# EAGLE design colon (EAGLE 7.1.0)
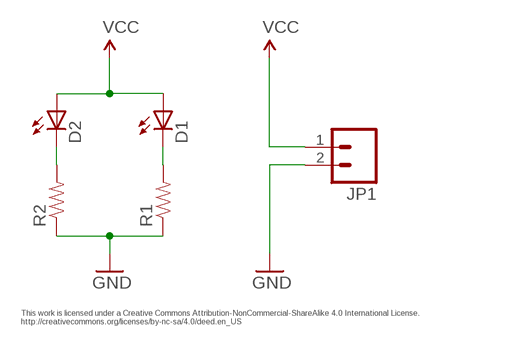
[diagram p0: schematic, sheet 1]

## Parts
D1  LED-RED1206  [LED-1206]
D2  LED-RED1206  [LED-1206]
JP1  M021X02_NO_SILK  [1X02_NO_SILK]
R1  RESISTOR0805-RES  [0805]
R2  RESISTOR0805-RES  [0805]

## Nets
GND: JP1.2 R1.1 R2.1
N$1: D2.C R2.2
N$2: D1.C R1.2
VCC: D1.A D2.A JP1.1

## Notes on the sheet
- This work is licensed under a Creative Commons Attribution-NonCommercial-ShareAlike 4.0 International License.
  http://creativecommons.org/licenses/by-nc-sa/4.0/deed.en_US

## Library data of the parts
D1 D2 = SparkFun-LED:LED-RED: Assorted Red LEDs; PROD_ID: DIO-00809; VALUE: RED
JP1 = SparkFun-Connectors:M02: Standard 2-pin 0.1" header. Use with
R1 R2 = SparkFun-Resistors:RESISTOR: Resistor

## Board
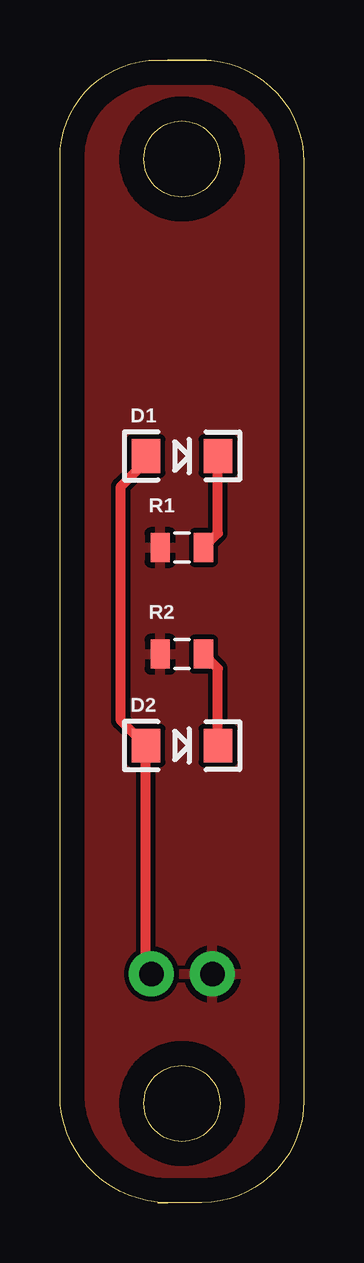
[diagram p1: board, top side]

Size 10.16 x 47.62 mm. Coordinates in mm from the lower left corner, seen from the top.
Outline: 4.49,0 5.9,0 arc90 10.16,4.26 10.16,43.37 arc90 5.9,47.62 4.07,47.62 arc90 0,43.56 0,43.18 0,42.55 0,4.49 arc90 4.49,0
Outline: 4.07,0 4.49,0
Outline: 6.09,47.62 4.49,47.62
Outline: 5.08,45.09 arc-180 5.08,41.91 arc-180 5.08,45.09
Outline: 5.08,2.54 arc-180 5.08,5.71 arc-180 5.08,2.54
Copper layers (1*16): Top 0.035mm / dielectric 1.5mm / Bottom 0.035mm
Design rules "default": minimum track width 10mil, minimum drill 24mil, track to track 8mil, track to pad 8mil, pad to pad 8mil, via to via 8mil, smd to smd 8mil, copper to edge 40mil, drill to drill 8mil, minimum pad ring 10mil, minimum via ring 8mil, stop-mask expansion 4mil, vias tented up to drill 0mil, thermal gap 10mil

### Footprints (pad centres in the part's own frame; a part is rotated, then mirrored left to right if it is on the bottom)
LED-1206 = smd 1.2 x 1.4: A -1.5,0; C 1.5,0
1X02_NO_SILK = drill 1.016 pad 1.88: 1 0,0; 2 2.54,0
0805 = smd 0.8 x 1.2: 1 -0.9,0; 2 0.9,0

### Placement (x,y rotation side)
D1  5.08,31.12 0 top
D2  5.08,19.05 0 top
JP1  3.81,9.53 0 top
R1  5.08,27.3 0 top
R2  5.08,22.86 0 top

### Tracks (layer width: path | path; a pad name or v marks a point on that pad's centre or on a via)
GND
  pour Top: -5.08,50.8 13.97,50.8 13.97,-3.17 -5.08,-3.17
N$1
  Top 0.406: D2.C 6.58,22.26 R2.2
N$2
  Top 0.406: R1.2 6.58,27.91 D1.C
VCC
  Top 0.406: JP1.1 3.58,9.75 D2.A 2.54,20.09 2.54,29.85 3.58,30.89 D1.A

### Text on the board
Unrouted: This work is licensed under a Creative Commons Attribution-NonCommercial-ShareAlike 4.0 International License. / http://creativecommons.org/licenses/by-nc-sa/4.0/deed.en_US
bNames: Kevin Rye, 2015 - V1.0 | Vcc | GND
